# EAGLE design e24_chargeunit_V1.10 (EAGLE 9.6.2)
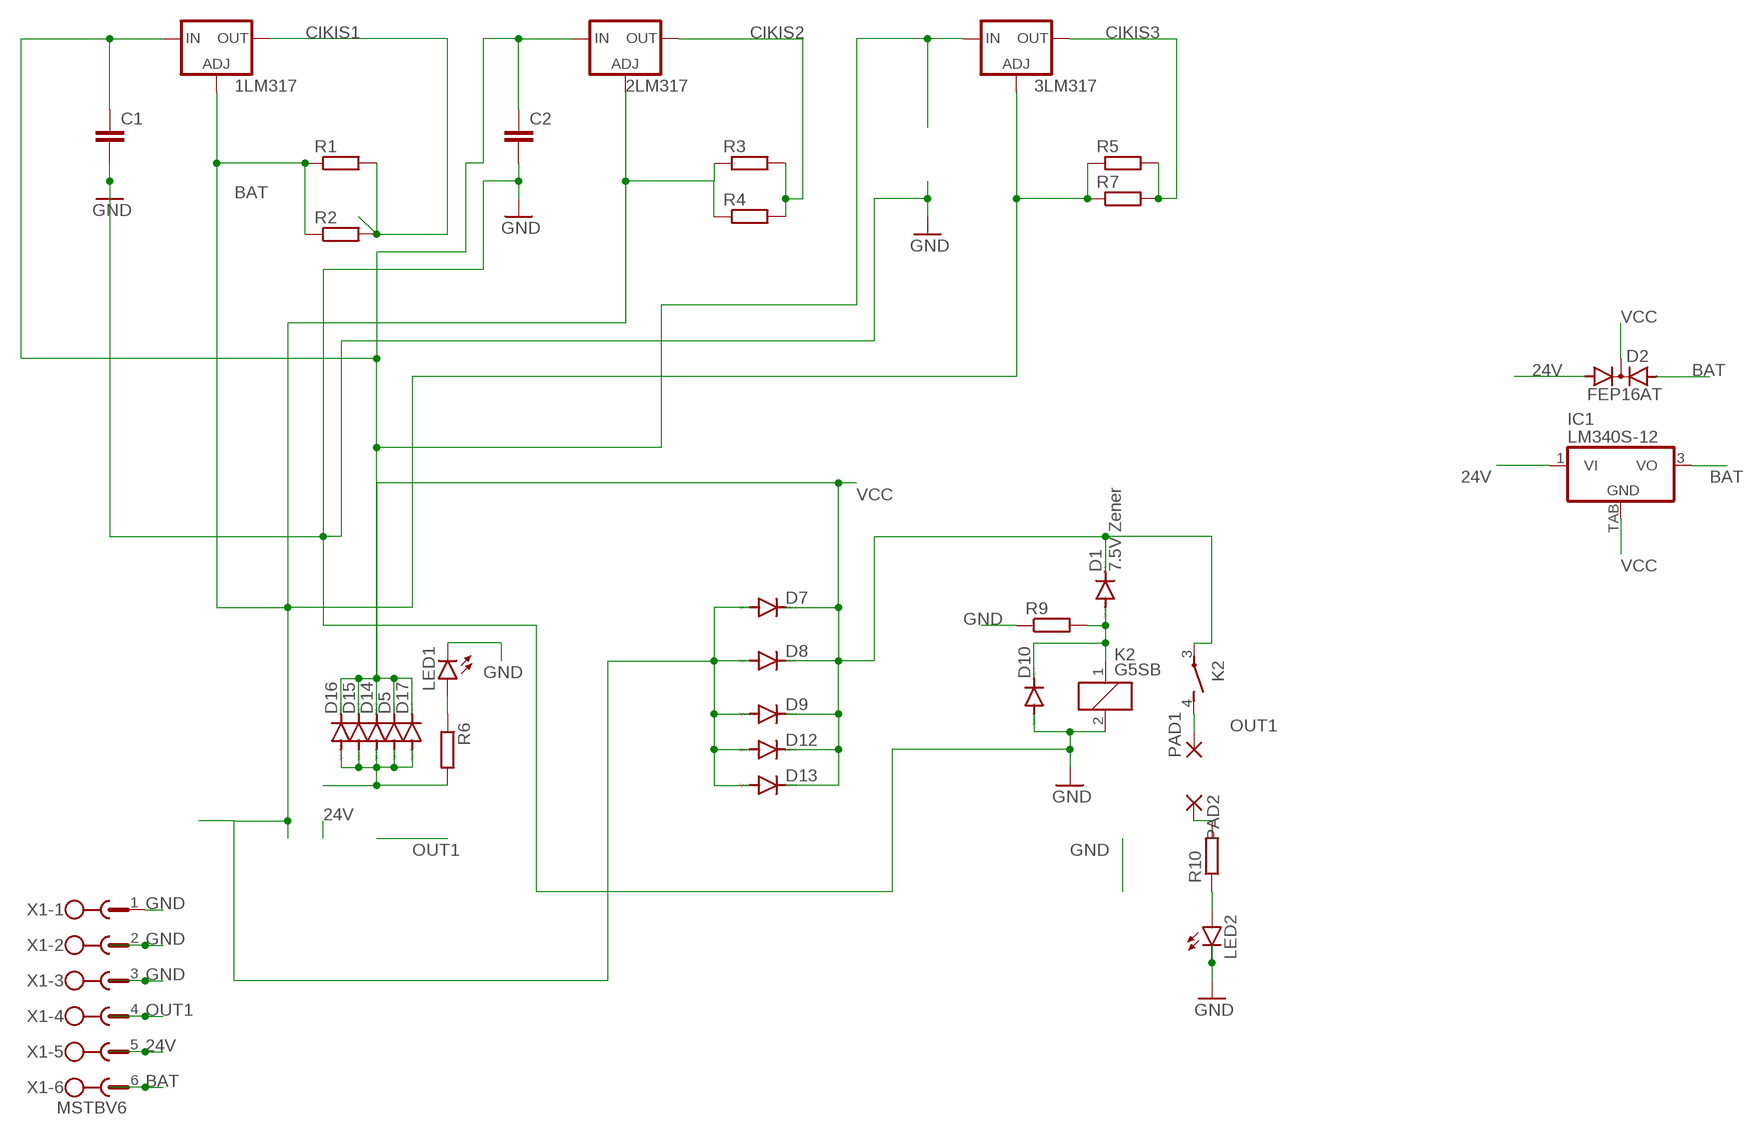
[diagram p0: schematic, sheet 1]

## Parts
1LM317  LM317TS  [317TS]
2LM317  LM317TS  [317TS]
3LM317  LM317TS  [317TS]
C1  C-EUC1206K  [C1206K]
C2  C-EUC1206K  [C1206K]
D1  7.5V Zener  DIODE-DO214AA  [DO214AA]
D2  FEP16AT  [TO220ABS]
D5  DIODE-DO214AA  [DO214AA]
D7  DIODE-DO214AA  [DO214AA]
D8  DIODE-DO214AA  [DO214AA]
D9  DIODE-DO214AA  [DO214AA]
D10  DIODE-DO214AA  [DO214AA]
D12  DIODE-DO214AA  [DO214AA]
D13  DIODE-DO214AA  [DO214AA]
D14  DIODE-DO214AA  [DO214AA]
D15  DIODE-DO214AA  [DO214AA]
D16  DIODE-DO214AA  [DO214AA]
D17  DIODE-DO214AA  [DO214AA]
IC1  LM340S-12  [TO263-3]
K2  G5SB  [G5SB]
LED1  LED3MM  [LED3MM]
LED2  LED3MM  [LED3MM]
PAD1  3,81/1,4  [3,81/1,4]
PAD2  3,81/1,4  [3,81/1,4]
R1  R-EU_R2512  [R2512]
R2  R-EU_R2512  [R2512]
R3  R-EU_R2512  [R2512]
R4  R-EU_R2512  [R2512]
R5  R-EU_R2512  [R2512]
R6  R-EU_M1206  [M1206]
R7  R-EU_R2512  [R2512]
R9  R-EU_M1206  [M1206]
R10  R-EU_M1206  [M1206]
X1  MSTBV6  [MSTBV6]

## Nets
24V: D2.A1 D5.A D14.A D15.A D16.A D17.A IC1.1(VI) R6.2 X1.5
BAT: 1LM317.1(ADJ) 2LM317.1(ADJ) 3LM317.1(ADJ) D2.A2 D7.A D8.A D9.A D12.A D13.A IC1.3(VO) R1.1 R2.1 R3.1 R4.1 R5.1 R7.1 X1.6
CIKIS1: 1LM317.2(OUT) R1.2 R2.2
CIKIS2: 2LM317.2(OUT) R3.2 R4.2
CIKIS3: 3LM317.2(OUT) R5.2 R7.2
GND: C1.2 C2.2 D10.A K2.2 LED1.K(C) LED2.K(C) R9.1 X1.1 X1.2 X1.3
N$5: PAD2.1(P) R10.2
N$9: LED1.A R6.1
N$12: D1.A D10.C K2.1 R9.2
N$13: LED2.A R10.1
OUT1: K2.4(S) PAD1.1(P) X1.4
VCC: 1LM317.3(IN) 2LM317.3(IN) 3LM317.3(IN) C1.1 C2.1 D1.C D2.C D5.C D7.C D8.C D9.C D12.C D13.C D14.C D15.C D16.C D17.C IC1.TAB(GND) K2.3(P)

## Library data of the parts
1LM317 2LM317 3LM317 = v-reg:LM317TS: VOLTAGE REGULATOR
C1 C2 = rcl:C-EU: CAPACITOR, European symbol; SPICEPREFIX: C
D1 D5 D7-D10 D12-D17 = diode:DIODE-: DIODE
D2 = diode:FEP16AT: DIODE dual ultra-fast recovery rectifier, common cathode
IC1 = linear:LM340?-*: Positive VOLTAGE REGULATOR Source: http://cache.national.com/ds/LM/LM340.pdf
K2 = said-relay1:G5SB: Compact Single-pole Relay for Switching 5 A Source: http://www.omron.com/ecb/products/pry/121/g5sb.html; OC_FARNELL: unknown; OC_NEWARK: unknown
LED1 LED2 = led:LED: LED
PAD1 PAD2 = wirepad:3,81/1,4: THROUGH-HOLE PAD
R1-R7 R9 R10 = rcl:R-EU_: RESISTOR, European symbol; SPICEPREFIX: R
X1 = con-phoenix-508:MSTBV6: PHOENIX; MPN: MSTBV 2,5/6-GF-5.08; OC_FARNELL: 1792796; OC_NEWARK: 69R9849

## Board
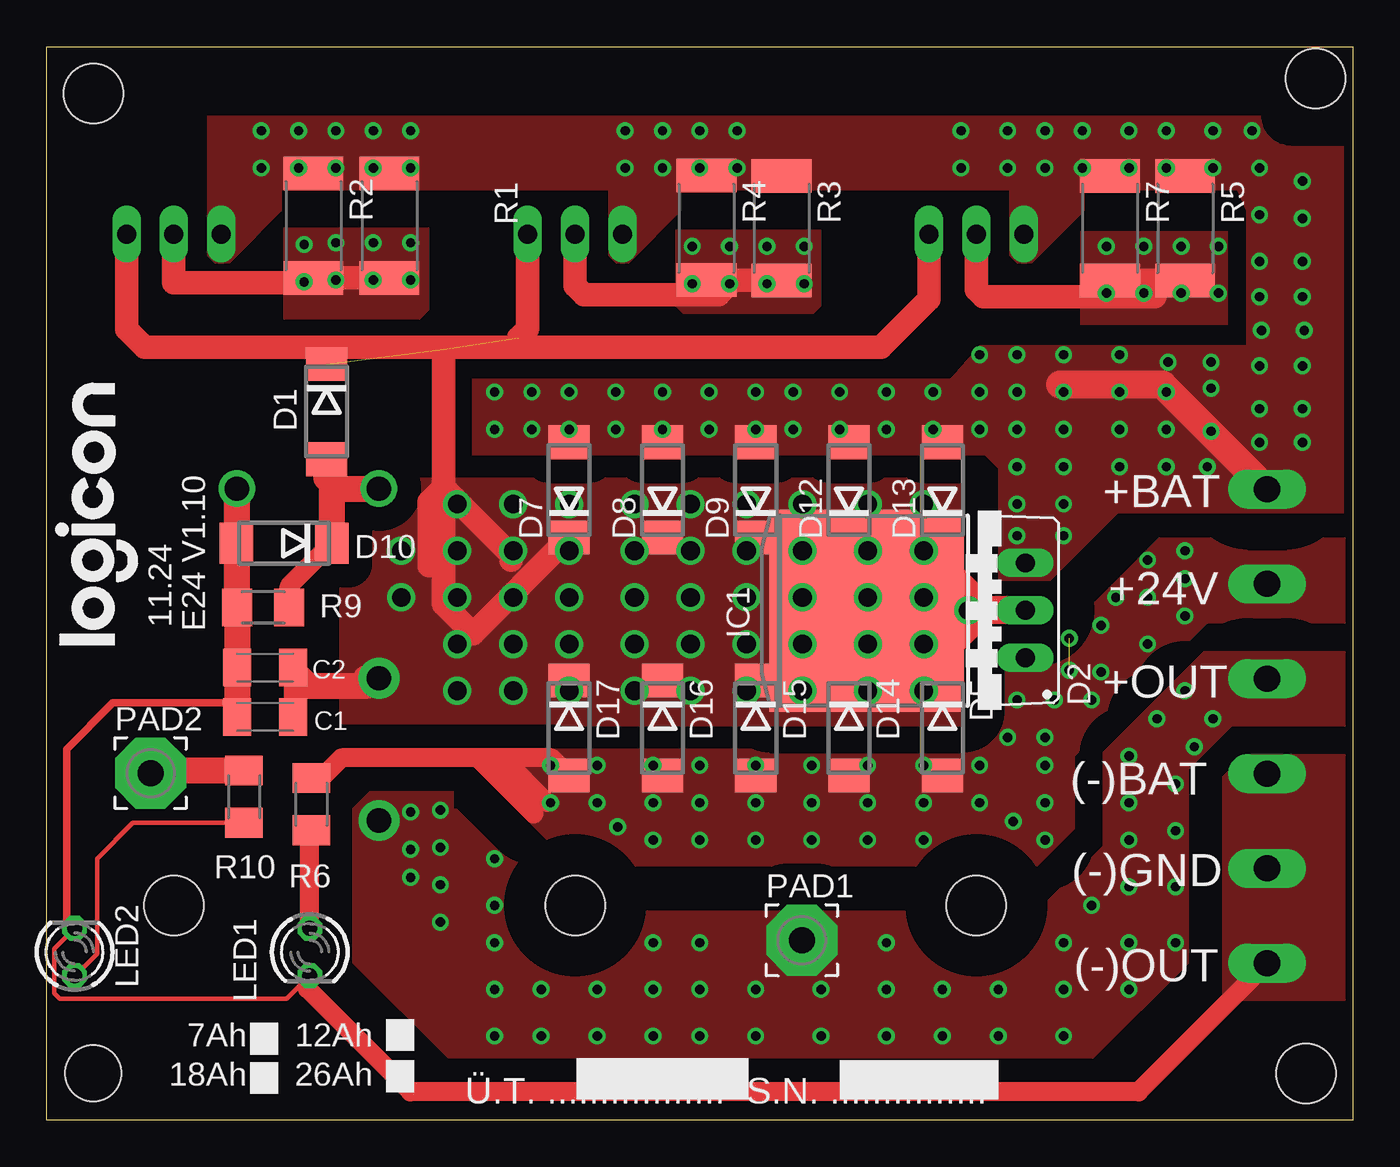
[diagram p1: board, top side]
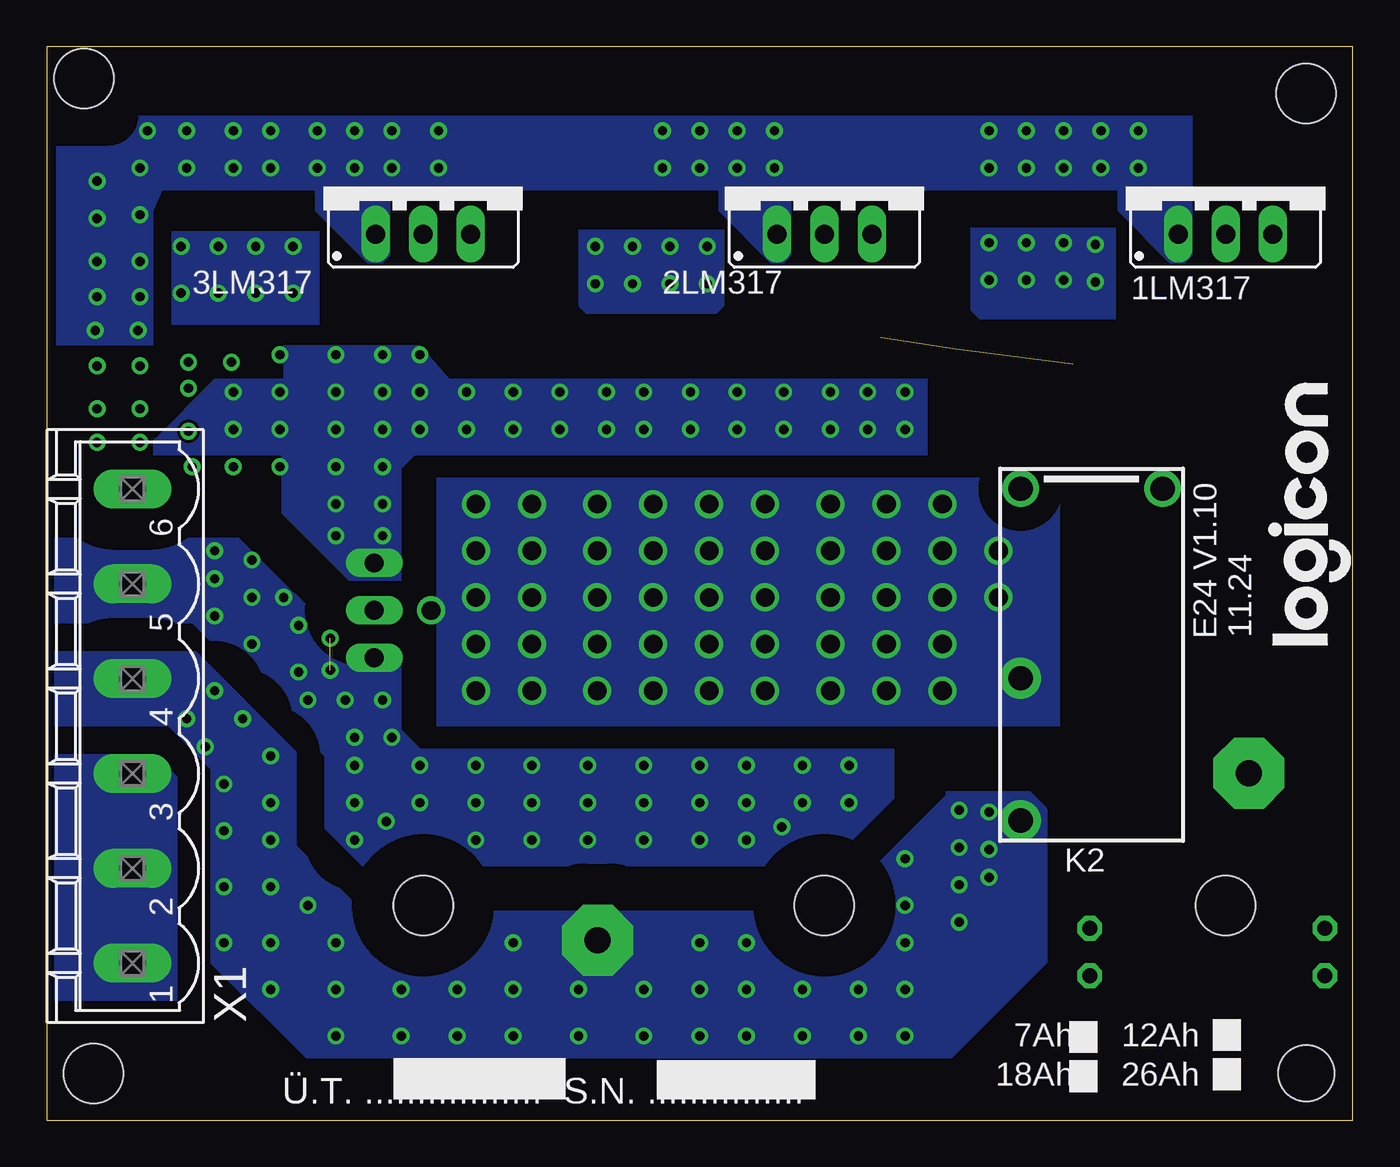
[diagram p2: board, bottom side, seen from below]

Size 70 x 57.5 mm. Coordinates in mm from the lower left corner, seen from the top.
Outline: 0,0 0,57.5 70,57.5 70,0 0,0
Copper layers (1*16): Top 0.035mm / dielectric 1.5mm / Bottom 0.035mm
Design rules "default *": minimum track width 6mil, minimum drill 0.35mm, track to track 6mil, track to pad 6mil, pad to pad 6mil, via to via 6mil, smd to smd 6mil, copper to edge 0mil, drill to drill 6mil, minimum pad ring 10mil, minimum via ring 8mil, stop-mask expansion 4mil, vias tented up to drill 0mil, thermal gap 10mil
Holes 3.2 mm at 6.82,11.5 28.32,11.5 49.82,11.5 2.5,55 68,55.8 67.5,2.5
Holes 3 mm at 2.5,2.5

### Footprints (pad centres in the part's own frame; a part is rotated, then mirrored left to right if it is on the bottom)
317TS = drill 1.016 long: 1 -2.54,-2.54; 2 0,-2.54; 3 2.54,-2.54
C1206K = smd 1.5 x 2: 1 -1.5,0; 2 1.5,0
DO214AA = smd 1.8 x 2.2: A 2.55,0; C -2.55,0
TO220ABS = drill 1.016 long: A1 -2.54,-2.54; A2 2.54,-2.54; C 0,-2.54
TO263-3 = smd 1.067 x 2.159: 1 -2.54,-5.791; 2 0,-5.791; 3 2.54,-5.791 | smd 10.8 x 10.41: TAB 0,2.54
G5SB = drill 1.3 pad 1.93: 1 7.62,3.81; 2 7.62,-3.81 | drill 1.3 pad 2.184: 3 -2.54,3.81; 4 -10.16,3.81
LED3MM = drill 0.813 octagon: A -1.27,0; K 1.27,0
3,81/1,4 = drill 1.397 pad 3.81 octagon: 1 0,0
R2512 = smd 1.8 x 3.2: 1 -2.8,0; 2 2.8,0
M1206 = smd 1.6 x 2: 1 -1.4,0; 2 1.4,0
MSTBV6 = drill 1.397 long: 1 -12.7,0; 2 -7.62,0; 3 -2.54,0; 4 2.54,0; 5 7.62,0; 6 12.7,0

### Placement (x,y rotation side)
1LM317  6.82,50 0 bottom
2LM317  28.32,50 0 bottom
3LM317  49.82,50 0 bottom
C1  11.71,21.59 180 top
C2  11.71,24.24 180 top
D1  15,37.95 270 top
D2  49.9,27.3 90 top
D5  48,21 270 top
D7  28,33.76 90 top
D8  33,33.76 90 top
D9  38,33.76 90 top
D10  12.73,30.9 180 top
D12  43,33.76 90 top
D13  48,33.76 90 top
D14  43,21 270 top
D15  38,21 270 top
D16  33,21 270 top
D17  28,21 270 top
IC1  46.48,27.28 90 top
K2  14,26.2 90 bottom
LED1  14.1,9 270 top
LED2  1.5,9 90 top
PAD1  40.47,9.63 0 top
PAD2  5.57,18.58 0 top
R1  18.37,47.91 270 top
R2  14.3,47.91 270 top
R3  39.38,47.78 270 top
R4  35.36,47.79 270 top
R5  61.01,47.77 270 top
R6  14.19,16.92 90 top
R7  56.98,47.78 270 top
R9  11.6,27.45 0 top
R10  10.58,17.32 90 top
X1  65.4,21.1 90 bottom

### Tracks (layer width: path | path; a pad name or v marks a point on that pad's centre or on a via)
24V  (via drill 0.5)  (1 unrouted)
  Top 1.016: D17.A 27.05,19.4 23.1,19.4 | R6.2 14.72,18.32 15.8,19.4 23.1,19.4 | 24.1,19.4 24.4,19.4 26.8,17 | 23.1,19.4 26.1,16.4
  other vias: 61,30.5 61,29 61,27 59,30 59,28 59,25.5 57.3,28 56.5,26.5 56.5,24 52,22.5 54,22.5 56,22.5 51.5,20.5 53.5,20.5 50,19 50,17 51.8,16 47,19 47,17 47,15 53.5,19 53.5,17 53.5,15 44,19 44,17 44,15 41,15 41,17 41,19 38,19 38,17 38,15 35,15 35,17 35,19 32.5,19 32.5,17 32.5,15 29.5,19 29.5,17 30.6,15.7 27,17 27,19 54.8,25.8 54.8,24.1
  pour Top (isolate 2.2, no thermals): 52.8,19.9 52.8,13.6 28.2,13.6 22.6,19.2 22.6,19.9
  pour Top (isolate 2.2, no thermals): 49.3,13.6 49.3,19.2 51,20.9 51,25.5 53.9,25.5 59.6,31.2 69.6,31.2 69.6,26.6 62.2,26.6 55.1,19.5 55.1,15.6 53.1,13.6
  pour Bottom (isolate 2.2, no thermals): 52.8,19.9 52.8,13.6 28.2,13.6 24.6,17.2 24.6,19.9
  pour Bottom (isolate 2.2, no thermals): 49.3,13.6 49.3,19.2 51,20.9 51,25.3 53.8,25.3 59.7,31.2 69.6,31.2 69.6,26.6 62.2,26.6 55.1,19.5 55.1,15.6 53.1,13.6
BAT  (via drill 0.5)
  Top 1.27: R3.1 | R5.1
  Top 1.5: X1.6 59.8,39.4 54.3,39.4
  other vias: 67.3,46 60,39 60,37 60,35 57.5,41 57.5,39 57.5,37 57.5,35 54.5,41 54.5,39 54.5,37 54.5,35 52,35 52,37 52,39 52,41 50,41 50,39 50,37 47.5,39 47.5,37 45,39 45,37 42.5,39 42.5,37 40,39 38,39 35.5,39 33,39 30.5,39 28,39 26,39 24,39 24,37 40,37 26,37 28,37 54.5,33 52,33 30.5,37 33,37 35.5,37 38,37 67.3,48.3 67.3,50.3 65,46 65,48.5 65,51 62.5,51 60,51 58,51 58,53 60,53 62.5,53 64.6,53 55.5,53 55.5,51 53.5,53 53.5,51 51.5,51 51.5,53 49,53 49,51 31,53 31,51 33,53 33,51 35,53 35,51 37,53 37,51 11.5,53 11.5,51 13.5,53 13.5,51 15.5,53 15.5,51 17.5,53 17.5,51 19.5,53 19.5,51 54.5,31.3 52,31.3 65,38.1 62.2,35 62.4,39.2 60.1,40.6 62.4,40.6 65,40.4 67.3,40.4 67.3,38.1 67.3,36.3 65,36.3 67.4,42.3 65.1,42.3 65,44.1 67.3,44.1
  pour Top (no thermals): 8.6,53.8 8.6,46.3 9,45.9 9.8,45.9 12.6,48.7 12.6,49.8 63.8,49.8 64.3,48.7 64.3,41.5 69.5,41.5 69.5,53.8
  pour Top (no thermals): 69.5,32.5 69.5,41.5 50,41.5 48,39.2 39.7,38.5 56.2,36.5 56.2,32.5
  pour Top (no thermals): 64.3,36.4 64.3,35.6 22.8,35.6 22.8,39.7 61,39.7
  pour Bottom (no thermals): 57.4,32.5 53.8,28.9 51,28.9 51,34.9 49.5,36.4 49.5,36.5 50.2,37.2 56.3,37.2 57.4,36.1
  pour Top (no thermals): 31,49.8 26.5,49.8 26.5,50.5 31,50.5
  pour Top (no thermals): 49.3,49.8 49.5,50 44.5,49.8
  pour Bottom (isolate 0.406, no thermals): 8.6,53.8 8.6,46.3 9,45.9 9.8,45.9 12.6,48.7 12.6,49.8 63.8,49.8 64.3,48.7 64.3,41.5 69.5,41.5 69.5,53.8
  pour Bottom (no thermals): 57.3,37.6 57.3,41.5 50,41.5 48,39.2 39.7,38.5 41.7,36.5 56.2,36.5
  pour Bottom (no thermals): 64.3,36.4 64.3,35.6 22.8,35.6 22.8,39.7 61,39.7
  pour Top (no thermals): 57.4,32.5 53.8,28.9 51,28.9 51,34.9 49.5,36.4 49.5,36.5 50.2,37.2 56.3,37.2 57.4,36.1
  pour Bottom (no thermals): 49.3,49.8 49.5,50 44.5,49.8
  pour Top (no thermals): 30.1,50.1 30.1,46.3 30.5,45.9 31.2,45.9 34,48.7 34,50.1
  pour Bottom (no thermals): 30.1,50.1 30.1,46.3 30.5,45.9 31.2,45.9 34,48.7 34,50.1
  pour Top (no thermals): 51.6,50 51.6,46.3 52,45.9 52.8,45.9 55.6,48.7 55.6,50
  pour Bottom (no thermals): 51.6,50 51.6,46.3 52,45.9 52.8,45.9 55.6,48.7 55.6,50
  cutout Top (no thermals): 65.1,53.8 arc90 66.7,52.2 69.5,52.2 69.5,53.8
  cutout Bottom (no thermals): 65.1,53.8 arc90 66.7,52.2 69.5,52.2 69.5,53.8
CIKIS1  (via drill 0.5)
  Top 1.27: 1LM317.2 6.82,44.85 14.04,44.85 R2.2 R1.2
  other vias: 13.8,46.9 13.8,44.9 15.5,47 15.5,45 17.5,47 17.5,45 19.5,47 19.5,45
  pour Bottom (isolate 1.27, no thermals): 12.7,42.9 12.7,47.8 20.5,47.8 20.5,43.4 20,42.9
  pour Top (no thermals): 12.7,47.8 20.5,47.8 20.5,43.4 20,42.9 12.7,42.9
CIKIS2  (via drill 0.5)
  Top 1.27: R3.2 R4.2 34.79,44.99 v34.6,44.8 | 2LM317.2 28.32,44.68 28.8,44.2 36,44.2 v36.6,44.8
  other vias: 34.6,46.8 36.6,46.8 38.6,46.8 40.6,46.8 40.6,44.8 38.6,44.8
  pour Top (no thermals): 33.7,43.6 33.7,47.7 41.5,47.7 41.5,43.6 41.1,43.2 34.1,43.2
  pour Bottom (no thermals): 33.7,43.6 33.7,47.7 41.5,47.7 41.5,43.6 41.1,43.2 34.1,43.2
CIKIS3  (via drill 0.5)
  Top 1.27: R5.2 R7.2 56.8,44.8 | 3LM317.2 49.82,44.48 50.2,44.1 59.4,44.1
  other vias: 56.8,46.8 56.8,44.3 58.8,46.8 58.8,44.3 60.8,46.8 60.8,44.3 62.8,46.8 62.8,44.3
  pour Top (no thermals): 55.4,42.6 55.4,47.6 63.3,47.6 63.3,42.6
  pour Bottom (no thermals): 55.4,42.6 55.4,47.6 63.3,47.6 63.3,42.6
GND
  Top 0.254: LED2.K 0.4,9.17 0.4,6.8 0.7,6.5 12.87,6.5 13.98,7.62 LED1.K
  Top 0.406: 10.21,22.34 3.54,22.34 1.07,19.87 1.07,10.27 LED2.K 1.07,10.27 | 14.1,7.17 LED1.K
  Top 1.016: X1.1 58.51,1.51 19.5,1.51 13.98,7.03 13.98,7.62 | C2.2 10.21,22.34
  Top 1.4: K2.2 D10.A 10.18,27.47 R9.1 C2.2 C1.2
  pour Top (no thermals): 64.2,19.6 69.6,19.6 69.6,6.4 63,6.4 63,18.4
  pour Bottom (no thermals): 64.2,19.6 69.6,19.6 69.6,6.4 63,6.4 63,18.4
N$2  (via drill 0.5)
  other vias: 62.4,36.9
N$5
  Top 1.4: PAD2.1 5.71,18.72 R10.2
N$9
  Top 1.016: LED1.A 14.1,15.52 R6.1
  Top 1.4: R6.1
N$12
  Top 1.016: R9.2 13,28.62 D10.C
  Top 1.4: D10.C 15.28,35.12 D1.A 15,34.4 15.58,33.82 K2.1
N$13
  Top 0.254: R10.1 4.62,15.92 2.7,14 2.7,8.9 1.53,7.73 LED2.A
  Top 1.4: R10.1
OUT1  (via drill 0.5)
  other vias: 19.5,13 19.5,16.5 19.5,14.5 21.1,16.6 21.1,14.6 21.1,12.6 21.1,10.6 24,14 24,11.5 24,9.5 24,7 24,4.5 26.5,7 26.5,4.5 29.5,7 29.5,4.5 32.5,9.5 32.5,7 32.5,4.5 35,9.5 35,7 35,4.5 45,9.5 45,7 45,4.5 48,7 48,4.5 51,7 51,4.5 54.5,9.5 54.5,7 54.5,4.5 58,12.5 58,9.5 58,7 56,11.5 58,19.5 58,17 58,15 61,23 62.5,21.5 59.5,21.5 61.5,20 60.5,18 60.5,15.5 60.5,12.5 60.5,9.5 38,7 38,4.5 41.5,7 41.5,4.5
  pour Top (isolate 2.2, no thermals): 21.8,17.6 28.2,11.2 53.1,11.2 56.6,14.7 56.6,6.1 21.8,6.1
  pour Top (no thermals): 16.4,8.4 16.4,16.7 17.3,17.6 21.8,17.6 21.8,6.1 56.6,6.1 56.6,19.7 62,25.1 69.6,25.1 69.6,21.1 63.5,21.1 61.2,18.8 61.2,8.4 56.1,3.3 21.5,3.3
  pour Bottom (isolate 2.2, no thermals): 21.8,17.4 28,11.2 53.1,11.2 56.6,14.7 56.6,6.1 21.8,6.1
  pour Bottom (no thermals): 16.4,8.4 16.4,16.7 17.3,17.6 21.8,17.6 21.8,6.1 56.6,6.1 56.6,19.7 62,25.1 69.6,25.1 69.6,21.1 63.5,21.1 61.2,18.8 61.2,8.4 56.1,3.3 21.5,3.3
VCC  (via drill 1, 1 pad 1.2)  (2 unrouted)
  Top 0.2: D1.C 15.9,41.4 16.5,41.4
  Top 1.016: C2.1 C1.1
  Top 1.27: 15.7,41.4 16.5,41.4 44.7,41.4 47.28,43.98 3LM317.3 | 1LM317.3 4.28,42.37 5.25,41.4 15.7,41.4 | 21.28,33.9 21.28,27.63 22.85,26.06 D7.C | 21.28,33.9 21.28,41.3 | 21.28,33.9 24.9,30.28 24.9,30 | 21.28,33.9 20.5,33.12 20.5,29.7 | 48,29.8 50.5,27.3 D2.C 50.4,27.3 48.5,25.4 | 25.3,41.9 25.78,42.38 2LM317.3 | D1.C 15,40.7 15.7,41.4
  Top 1.4: K2.3 17.11,23.66 17.11,23.24 14.01,23.24 13.21,24.04 C2.1
  Top 1.5: D2.C 44.1,27.3 43.4,26.6 | D2.C 49.5,27.3 47.5,29.3 | D2.C 49.8,27.3 48.6,26.1
  other vias: 47,33 47,30.5 47,28 47,25.5 47,23 44,23 44,25.5 44,28 44,30.5 44,33 40.5,33 40.5,30.5 40.5,28 40.5,25.5 40.5,23 37.5,33 37.5,30.5 37.5,28 37.5,25.5 37.5,23 34.5,23 34.5,25.5 34.5,28 34.5,30.5 34.5,33 31.5,33 31.5,30.5 31.5,28 31.5,25.5 31.5,23 28,23 28,25.5 28,28 28,30.5 28,33 25,23 25,25.5 25,28 25,30.5 25,33 22,33 22,30.5 22,28 22,25.5 22,23 19,30.5 19,28 49.4,27.3
  pour Top (isolate 1.27, no thermals): 49.1,34.4 15.7,34.4 15.7,21.1 49.1,21.1
  pour Bottom (isolate 1.27, no thermals): 49.1,34.4 15.7,34.4 15.7,21.1 49.1,21.1

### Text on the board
tPlace: +BAT | +24V | 11.24 | E24 V1.10 | +OUT | (-)BAT | (-)GND | (-)OUT | 7Ah 12Ah | 18Ah 26Ah | Ü.T. ................. S.N. ...............
bPlace: 11.24 | E24 V1.10 | 7Ah 12Ah | 18Ah 26Ah | Ü.T. ................. S.N. ...............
